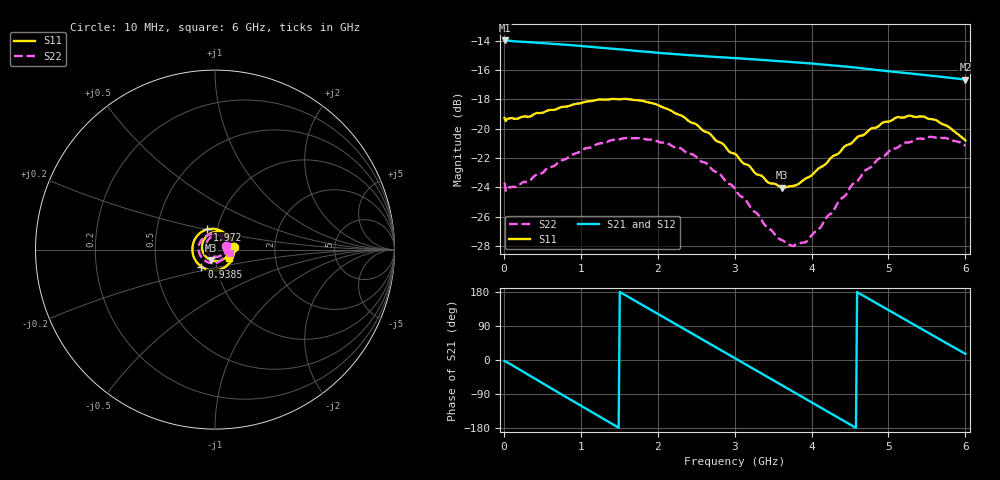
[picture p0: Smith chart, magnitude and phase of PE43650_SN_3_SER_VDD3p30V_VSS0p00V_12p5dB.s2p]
!Keysight Technologies,N5245B,MY57181451,A.13.50.07
!Date: Tuesday, May 07, 2019 08:00:10
!Correction: S11(Full 2 Port(1,2))
!S21(Full 2 Port(1,2))
!S12(Full 2 Port(1,2))
!S22(Full 2 Port(1,2))
!S2P File: Measurements: S11, S21, S12, S22:
# Hz S  dB  R 50
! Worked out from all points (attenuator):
!   401 points, 10 MHz to 6 GHz, reference 50 ohm
!   highest |S21| = -13.97 dB at 10 MHz (marker M1); lowest = -16.6 dB at 6 GHz (marker M2)
!   lowest |S11| = -24.0 dB at 3.619 GHz (marker M3), VSWR 1.13, Z = 47.7 - j5.69 ohm
!   |S11| at or under -10 dB: start of sweep to end of sweep
!   |S22| runs from -28.0 to -20.5 dB; largest |S21 - S12| = 0.0015
!   S11 on the Smith chart (normalised r, x): 10 MHz: 1.24, +0.03; 938.5 MHz: 0.85, -0.16; 1.972 GHz: 0.89, +0.20; 6 GHz: 1.16, -0.11
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1e7  -19.27 6.9  -13.97 -3.1  -13.98 -3.5  -23.69 16.4
2.496e8  -19.17 -36.5  -14.06 -30.7  -14.11 -30.8  -23.66 -36.8
5.1915e8  -18.88 -74.1  -14.15 -63.2  -14.20 -63.1  -22.94 -75.5
9.3845e8  -18.30 -128.3  -14.32 -113.2  -14.37 -113.2  -21.68 -127.6
1.013325e9  -18.23 -137.7  -14.36 -122.0  -14.40 -122.1  -21.48 -136.7
1.2679e9  -18.00 -167.9  -14.46 -152.2  -14.52 -152.2  -20.99 -164.6
1.492525e9  -17.98 165.8  -14.56 -178.7  -14.63 -178.6  -20.74 171.3
1.71715e9  -18.04 140.3  -14.68 154.9  -14.74 154.9  -20.65 148.2
1.971725e9  -18.31 112.0  -14.79 125.2  -14.85 125.2  -20.81 122.5
2.01665e9  -18.42 107.0  -14.81 119.9  -14.86 119.9  -20.91 117.9
2.241275e9  -18.97 81.5  -14.91 93.7  -14.96 93.7  -21.28 94.7
2.4659e9  -19.62 55.2  -14.99 67.5  -15.05 67.6  -21.79 71.8
2.750425e9  -20.78 21.3  -15.09 34.3  -15.15 34.4  -22.94 40.8
3.005e9  -21.73 -12.7  -15.17 4.6  -15.22 4.7  -24.12 11.6
3.289525e9  -23.12 -54.6  -15.27 -28.6  -15.32 -28.5  -25.78 -27.4
3.618975e9  -24.03 -109.0  -15.39 -67.1  -15.44 -67.1  -27.63 -80.9
3.7837e9  -23.88 -137.4  -15.46 -86.4  -15.51 -86.3  -27.93 -111.4
4.008325e9  -23.14 -174.1  -15.54 -112.6  -15.59 -112.6  -27.24 -152.4
4.517475e9  -20.99 116.1  -15.79 -172.2  -15.84 -172.1  -23.89 132.6
5.01165e9  -19.50 60.8  -16.07 130.4  -16.12 130.5  -21.51 78.2
5.475875e9  -19.20 14.7  -16.32 76.6  -16.38 76.8  -20.68 33.7
6e9  -20.81 -32.6  -16.63 16.2  -16.69 16.2  -21.17 -11.7
